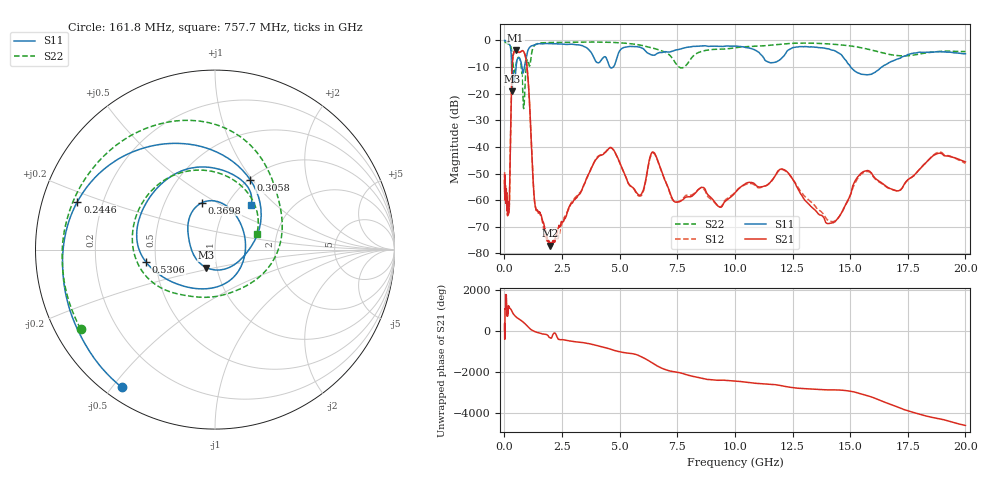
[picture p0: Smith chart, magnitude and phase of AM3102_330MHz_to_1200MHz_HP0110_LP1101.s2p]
! Date/Time: Tue, Sep 11, 2018 5:15 PM
! Network Analyzer: Agilent Technologies E8362B Rev: A.07.50.63
! Sweep from 0.010 to 20.000 GHz, 1601 Points, Sweep Type: LOG
! Power Supply: 4.949 V, 0.001 A
# Hz S DB R 50
!freq MagS11 AngS11 MagS21 AngS21 MagS12 AngS12 MagS22 AngS22
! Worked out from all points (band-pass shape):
!   1601 points, 10 MHz to 20 GHz, reference 50 ohm
!   highest |S21| = -3.61 dB at 487.1 MHz (marker M1); lowest = -77.0 dB at 1.988 GHz (marker M2)
!   |S21| within 3 dB of the highest: 363.7 MHz to 929.1 MHz (565.4 MHz wide, 87.5 % of centre)
!   lowest |S11| = -19.1 dB at 337.9 MHz (marker M3), VSWR 1.25, Z = 44.5 - j9.02 ohm
!   |S11| at or under -10 dB: 314.8 MHz to 507.9 MHz (193.1 MHz wide, 46.9 % of centre); 4.581 GHz to 4.719 GHz (137.8 MHz wide, 2.96 % of centre); 15.03 GHz to 16.37 GHz (1.344 GHz wide, 8.56 % of centre)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
!   |S22| runs from -25.6 to -0.3 dB; largest |S21 - S12| = 0.011
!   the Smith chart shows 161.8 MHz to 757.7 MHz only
!   S11 on the Smith chart (normalised r, x): 161.8 MHz: 0.05, -0.53; 244.6 MHz: 0.11, +0.17; 305.8 MHz: 1.02, +0.98; 369.8 MHz: 0.76, +0.43; 530.6 MHz: 0.44, -0.07; 757.7 MHz: 1.28, +0.71
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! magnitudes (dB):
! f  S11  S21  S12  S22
! 10 MHz  0.0  -52.5  -49.4  -0.3
! 35.55 MHz  0.0  -57.3  -59.0  -0.6
! 126.4 MHz  -0.4  -63.4  -60.9  -1.1
! 161.8 MHz  -0.7  -62.1  -62.6  -1.2
! 244.6 MHz  -1.8  -47.8  -47.8  -1.7
! 305.8 MHz  -7.2  -19.0  -19.0  -3.2
! 337.9 MHz  -19.1  -9.5  -9.5  -5.9
! 369.8 MHz  -11.3  -6.2  -6.3  -8.4
! 447.2 MHz  -14.7  -3.8  -3.8  -11.6
! 487.1 MHz  -12.1  -3.6  -3.7  -10.2
! 530.6 MHz  -8.1  -3.9  -4.0  -7.8
! 757.7 MHz  -9.9  -3.9  -3.9  -12.1
! 841.2 MHz  -11.4  -4.2  -4.3  -25.5
! 988.7 MHz  -4.6  -10.5  -10.6  -7.4
! 1.302 GHz  -1.6  -59.7  -60.0  -1.9
! 1.59 GHz  -1.3  -65.5  -66.0  -0.9
! 1.988 GHz  -1.2  -77.0  -76.5  -0.8
! 4.5 GHz  -8.3  -40.9  -40.8  -0.6
! 5.652 GHz  -2.3  -56.0  -56.3  -1.4
! 12.09 GHz  -6.1  -48.4  -48.5  -1.3
! 14.14 GHz  -3.4  -68.6  -67.9  -1.3
! 20 GHz  -5.0  -45.6  -46.2  -4.2
